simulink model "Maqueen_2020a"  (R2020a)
settings: Solver=VariableStepAuto  StartTime=0.0  StopTime=2  RelTol=1e-3
model workspace: external: MAT-File (data not in the file)
undefined symbols (not defined in the file or in its folder): deg, kg, m, mm, N, rad, s, smiData, X, Y, Z
libraries: sm_lib x459, fl_lib x12, nesl_utility x10
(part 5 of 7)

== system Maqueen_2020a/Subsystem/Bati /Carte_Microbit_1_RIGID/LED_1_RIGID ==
  ReferenceFrame : sm_lib/Frames and Transforms/Reference Frame
  Solid : sm_lib/Body Elements/File Solid  ExtGeomFileName=LED_Defaut_sldprt.STL  UnitType=Custom  ExtGeomFileUnits=mm  StepReaderType=HEX  ExportConvexHullGeometry=off  InertiaType=Custom  Mass=smiData.Solid(10).mass  MassUnits=kg  CenterOfMass=smiData.Solid(10).CoM  CenterOfMassUnits=mm  MomentsOfInertia=smiData.Solid(10).MoI  MomentsOfInertiaUnits=kg*mm^2  ProductsOfInertia=smiData.Solid(10).PoI  ProductsOfInertiaUnits=kg*mm^2  BasedOnType=Density  Density=1000  DensityUnits=kg/m^3  DoExposeReferenceFrame=on  SerializedFrames=<Frames/>  GraphicType=FromGeometry  MarkerShape=Sphere  MarkerSize=10  GraphicVisPropType=SimpleVisualProperties  GraphicDiffuseColor=smiData.Solid(10).color  GraphicSpecularColor=[0.5 0.5 0.5 1.0]  GraphicAmbientColor=[0.15 0.15 0.15 1.0]  GraphicEmissiveColor=[0.0 0.0 0.0 1.0]  GraphicShininess=75  GraphicOpacity=smiData.Solid(10).opacity
  F : PMIOPort  Side=Left
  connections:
  ReferenceFrame/RConn1 -- Solid/RConn1 -- F/RConn1

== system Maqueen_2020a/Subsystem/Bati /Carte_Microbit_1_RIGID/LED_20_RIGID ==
  ReferenceFrame : sm_lib/Frames and Transforms/Reference Frame
  Solid : sm_lib/Body Elements/File Solid  ExtGeomFileName=LED_Defaut_sldprt.STL  UnitType=Custom  ExtGeomFileUnits=mm  StepReaderType=HEX  ExportConvexHullGeometry=off  InertiaType=Custom  Mass=smiData.Solid(10).mass  MassUnits=kg  CenterOfMass=smiData.Solid(10).CoM  CenterOfMassUnits=mm  MomentsOfInertia=smiData.Solid(10).MoI  MomentsOfInertiaUnits=kg*mm^2  ProductsOfInertia=smiData.Solid(10).PoI  ProductsOfInertiaUnits=kg*mm^2  BasedOnType=Density  Density=1000  DensityUnits=kg/m^3  DoExposeReferenceFrame=on  SerializedFrames=<Frames/>  GraphicType=FromGeometry  MarkerShape=Sphere  MarkerSize=10  GraphicVisPropType=SimpleVisualProperties  GraphicDiffuseColor=smiData.Solid(10).color  GraphicSpecularColor=[0.5 0.5 0.5 1.0]  GraphicAmbientColor=[0.15 0.15 0.15 1.0]  GraphicEmissiveColor=[0.0 0.0 0.0 1.0]  GraphicShininess=75  GraphicOpacity=smiData.Solid(10).opacity
  F : PMIOPort  Side=Left
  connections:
  ReferenceFrame/RConn1 -- Solid/RConn1 -- F/RConn1

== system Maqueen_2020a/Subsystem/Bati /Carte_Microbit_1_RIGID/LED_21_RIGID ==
  ReferenceFrame : sm_lib/Frames and Transforms/Reference Frame
  Solid : sm_lib/Body Elements/File Solid  ExtGeomFileName=LED_Defaut_sldprt.STL  UnitType=Custom  ExtGeomFileUnits=mm  StepReaderType=HEX  ExportConvexHullGeometry=off  InertiaType=Custom  Mass=smiData.Solid(10).mass  MassUnits=kg  CenterOfMass=smiData.Solid(10).CoM  CenterOfMassUnits=mm  MomentsOfInertia=smiData.Solid(10).MoI  MomentsOfInertiaUnits=kg*mm^2  ProductsOfInertia=smiData.Solid(10).PoI  ProductsOfInertiaUnits=kg*mm^2  BasedOnType=Density  Density=1000  DensityUnits=kg/m^3  DoExposeReferenceFrame=on  SerializedFrames=<Frames/>  GraphicType=FromGeometry  MarkerShape=Sphere  MarkerSize=10  GraphicVisPropType=SimpleVisualProperties  GraphicDiffuseColor=smiData.Solid(10).color  GraphicSpecularColor=[0.5 0.5 0.5 1.0]  GraphicAmbientColor=[0.15 0.15 0.15 1.0]  GraphicEmissiveColor=[0.0 0.0 0.0 1.0]  GraphicShininess=75  GraphicOpacity=smiData.Solid(10).opacity
  F : PMIOPort  Side=Left
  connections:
  ReferenceFrame/RConn1 -- Solid/RConn1 -- F/RConn1

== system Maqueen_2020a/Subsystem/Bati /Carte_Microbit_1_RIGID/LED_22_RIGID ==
  ReferenceFrame : sm_lib/Frames and Transforms/Reference Frame
  Solid : sm_lib/Body Elements/File Solid  ExtGeomFileName=LED_Defaut_sldprt.STL  UnitType=Custom  ExtGeomFileUnits=mm  StepReaderType=HEX  ExportConvexHullGeometry=off  InertiaType=Custom  Mass=smiData.Solid(10).mass  MassUnits=kg  CenterOfMass=smiData.Solid(10).CoM  CenterOfMassUnits=mm  MomentsOfInertia=smiData.Solid(10).MoI  MomentsOfInertiaUnits=kg*mm^2  ProductsOfInertia=smiData.Solid(10).PoI  ProductsOfInertiaUnits=kg*mm^2  BasedOnType=Density  Density=1000  DensityUnits=kg/m^3  DoExposeReferenceFrame=on  SerializedFrames=<Frames/>  GraphicType=FromGeometry  MarkerShape=Sphere  MarkerSize=10  GraphicVisPropType=SimpleVisualProperties  GraphicDiffuseColor=smiData.Solid(10).color  GraphicSpecularColor=[0.5 0.5 0.5 1.0]  GraphicAmbientColor=[0.15 0.15 0.15 1.0]  GraphicEmissiveColor=[0.0 0.0 0.0 1.0]  GraphicShininess=75  GraphicOpacity=smiData.Solid(10).opacity
  F : PMIOPort  Side=Left
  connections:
  ReferenceFrame/RConn1 -- Solid/RConn1 -- F/RConn1

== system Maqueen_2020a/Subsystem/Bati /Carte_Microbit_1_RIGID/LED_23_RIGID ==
  ReferenceFrame : sm_lib/Frames and Transforms/Reference Frame
  Solid : sm_lib/Body Elements/File Solid  ExtGeomFileName=LED_Defaut_sldprt.STL  UnitType=Custom  ExtGeomFileUnits=mm  StepReaderType=HEX  ExportConvexHullGeometry=off  InertiaType=Custom  Mass=smiData.Solid(10).mass  MassUnits=kg  CenterOfMass=smiData.Solid(10).CoM  CenterOfMassUnits=mm  MomentsOfInertia=smiData.Solid(10).MoI  MomentsOfInertiaUnits=kg*mm^2  ProductsOfInertia=smiData.Solid(10).PoI  ProductsOfInertiaUnits=kg*mm^2  BasedOnType=Density  Density=1000  DensityUnits=kg/m^3  DoExposeReferenceFrame=on  SerializedFrames=<Frames/>  GraphicType=FromGeometry  MarkerShape=Sphere  MarkerSize=10  GraphicVisPropType=SimpleVisualProperties  GraphicDiffuseColor=smiData.Solid(10).color  GraphicSpecularColor=[0.5 0.5 0.5 1.0]  GraphicAmbientColor=[0.15 0.15 0.15 1.0]  GraphicEmissiveColor=[0.0 0.0 0.0 1.0]  GraphicShininess=75  GraphicOpacity=smiData.Solid(10).opacity
  F : PMIOPort  Side=Left
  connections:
  ReferenceFrame/RConn1 -- Solid/RConn1 -- F/RConn1

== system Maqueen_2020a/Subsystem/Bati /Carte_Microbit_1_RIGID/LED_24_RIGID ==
  ReferenceFrame : sm_lib/Frames and Transforms/Reference Frame
  Solid : sm_lib/Body Elements/File Solid  ExtGeomFileName=LED_Defaut_sldprt.STL  UnitType=Custom  ExtGeomFileUnits=mm  StepReaderType=HEX  ExportConvexHullGeometry=off  InertiaType=Custom  Mass=smiData.Solid(10).mass  MassUnits=kg  CenterOfMass=smiData.Solid(10).CoM  CenterOfMassUnits=mm  MomentsOfInertia=smiData.Solid(10).MoI  MomentsOfInertiaUnits=kg*mm^2  ProductsOfInertia=smiData.Solid(10).PoI  ProductsOfInertiaUnits=kg*mm^2  BasedOnType=Density  Density=1000  DensityUnits=kg/m^3  DoExposeReferenceFrame=on  SerializedFrames=<Frames/>  GraphicType=FromGeometry  MarkerShape=Sphere  MarkerSize=10  GraphicVisPropType=SimpleVisualProperties  GraphicDiffuseColor=smiData.Solid(10).color  GraphicSpecularColor=[0.5 0.5 0.5 1.0]  GraphicAmbientColor=[0.15 0.15 0.15 1.0]  GraphicEmissiveColor=[0.0 0.0 0.0 1.0]  GraphicShininess=75  GraphicOpacity=smiData.Solid(10).opacity
  F : PMIOPort  Side=Left
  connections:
  ReferenceFrame/RConn1 -- Solid/RConn1 -- F/RConn1

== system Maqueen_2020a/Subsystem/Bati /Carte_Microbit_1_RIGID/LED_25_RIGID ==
  ReferenceFrame : sm_lib/Frames and Transforms/Reference Frame
  Solid : sm_lib/Body Elements/File Solid  ExtGeomFileName=LED_Defaut_sldprt.STL  UnitType=Custom  ExtGeomFileUnits=mm  StepReaderType=HEX  ExportConvexHullGeometry=off  InertiaType=Custom  Mass=smiData.Solid(10).mass  MassUnits=kg  CenterOfMass=smiData.Solid(10).CoM  CenterOfMassUnits=mm  MomentsOfInertia=smiData.Solid(10).MoI  MomentsOfInertiaUnits=kg*mm^2  ProductsOfInertia=smiData.Solid(10).PoI  ProductsOfInertiaUnits=kg*mm^2  BasedOnType=Density  Density=1000  DensityUnits=kg/m^3  DoExposeReferenceFrame=on  SerializedFrames=<Frames/>  GraphicType=FromGeometry  MarkerShape=Sphere  MarkerSize=10  GraphicVisPropType=SimpleVisualProperties  GraphicDiffuseColor=smiData.Solid(10).color  GraphicSpecularColor=[0.5 0.5 0.5 1.0]  GraphicAmbientColor=[0.15 0.15 0.15 1.0]  GraphicEmissiveColor=[0.0 0.0 0.0 1.0]  GraphicShininess=75  GraphicOpacity=smiData.Solid(10).opacity
  F : PMIOPort  Side=Left
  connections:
  ReferenceFrame/RConn1 -- Solid/RConn1 -- F/RConn1

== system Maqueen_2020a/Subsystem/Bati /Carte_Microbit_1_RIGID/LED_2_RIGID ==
  ReferenceFrame : sm_lib/Frames and Transforms/Reference Frame
  Solid : sm_lib/Body Elements/File Solid  ExtGeomFileName=LED_Defaut_sldprt.STL  UnitType=Custom  ExtGeomFileUnits=mm  StepReaderType=HEX  ExportConvexHullGeometry=off  InertiaType=Custom  Mass=smiData.Solid(10).mass  MassUnits=kg  CenterOfMass=smiData.Solid(10).CoM  CenterOfMassUnits=mm  MomentsOfInertia=smiData.Solid(10).MoI  MomentsOfInertiaUnits=kg*mm^2  ProductsOfInertia=smiData.Solid(10).PoI  ProductsOfInertiaUnits=kg*mm^2  BasedOnType=Density  Density=1000  DensityUnits=kg/m^3  DoExposeReferenceFrame=on  SerializedFrames=<Frames/>  GraphicType=FromGeometry  MarkerShape=Sphere  MarkerSize=10  GraphicVisPropType=SimpleVisualProperties  GraphicDiffuseColor=smiData.Solid(10).color  GraphicSpecularColor=[0.5 0.5 0.5 1.0]  GraphicAmbientColor=[0.15 0.15 0.15 1.0]  GraphicEmissiveColor=[0.0 0.0 0.0 1.0]  GraphicShininess=75  GraphicOpacity=smiData.Solid(10).opacity
  F : PMIOPort  Side=Left
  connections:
  ReferenceFrame/RConn1 -- Solid/RConn1 -- F/RConn1

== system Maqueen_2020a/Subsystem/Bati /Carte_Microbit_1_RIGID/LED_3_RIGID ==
  ReferenceFrame : sm_lib/Frames and Transforms/Reference Frame
  Solid : sm_lib/Body Elements/File Solid  ExtGeomFileName=LED_Defaut_sldprt.STL  UnitType=Custom  ExtGeomFileUnits=mm  StepReaderType=HEX  ExportConvexHullGeometry=off  InertiaType=Custom  Mass=smiData.Solid(10).mass  MassUnits=kg  CenterOfMass=smiData.Solid(10).CoM  CenterOfMassUnits=mm  MomentsOfInertia=smiData.Solid(10).MoI  MomentsOfInertiaUnits=kg*mm^2  ProductsOfInertia=smiData.Solid(10).PoI  ProductsOfInertiaUnits=kg*mm^2  BasedOnType=Density  Density=1000  DensityUnits=kg/m^3  DoExposeReferenceFrame=on  SerializedFrames=<Frames/>  GraphicType=FromGeometry  MarkerShape=Sphere  MarkerSize=10  GraphicVisPropType=SimpleVisualProperties  GraphicDiffuseColor=smiData.Solid(10).color  GraphicSpecularColor=[0.5 0.5 0.5 1.0]  GraphicAmbientColor=[0.15 0.15 0.15 1.0]  GraphicEmissiveColor=[0.0 0.0 0.0 1.0]  GraphicShininess=75  GraphicOpacity=smiData.Solid(10).opacity
  F : PMIOPort  Side=Left
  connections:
  ReferenceFrame/RConn1 -- Solid/RConn1 -- F/RConn1

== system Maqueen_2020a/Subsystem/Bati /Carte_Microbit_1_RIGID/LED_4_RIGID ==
  ReferenceFrame : sm_lib/Frames and Transforms/Reference Frame
  Solid : sm_lib/Body Elements/File Solid  ExtGeomFileName=LED_Defaut_sldprt.STL  UnitType=Custom  ExtGeomFileUnits=mm  StepReaderType=HEX  ExportConvexHullGeometry=off  InertiaType=Custom  Mass=smiData.Solid(10).mass  MassUnits=kg  CenterOfMass=smiData.Solid(10).CoM  CenterOfMassUnits=mm  MomentsOfInertia=smiData.Solid(10).MoI  MomentsOfInertiaUnits=kg*mm^2  ProductsOfInertia=smiData.Solid(10).PoI  ProductsOfInertiaUnits=kg*mm^2  BasedOnType=Density  Density=1000  DensityUnits=kg/m^3  DoExposeReferenceFrame=on  SerializedFrames=<Frames/>  GraphicType=FromGeometry  MarkerShape=Sphere  MarkerSize=10  GraphicVisPropType=SimpleVisualProperties  GraphicDiffuseColor=smiData.Solid(10).color  GraphicSpecularColor=[0.5 0.5 0.5 1.0]  GraphicAmbientColor=[0.15 0.15 0.15 1.0]  GraphicEmissiveColor=[0.0 0.0 0.0 1.0]  GraphicShininess=75  GraphicOpacity=smiData.Solid(10).opacity
  F : PMIOPort  Side=Left
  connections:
  ReferenceFrame/RConn1 -- Solid/RConn1 -- F/RConn1

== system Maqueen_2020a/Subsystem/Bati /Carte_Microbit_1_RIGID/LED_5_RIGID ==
  ReferenceFrame : sm_lib/Frames and Transforms/Reference Frame
  Solid : sm_lib/Body Elements/File Solid  ExtGeomFileName=LED_Defaut_sldprt.STL  UnitType=Custom  ExtGeomFileUnits=mm  StepReaderType=HEX  ExportConvexHullGeometry=off  InertiaType=Custom  Mass=smiData.Solid(10).mass  MassUnits=kg  CenterOfMass=smiData.Solid(10).CoM  CenterOfMassUnits=mm  MomentsOfInertia=smiData.Solid(10).MoI  MomentsOfInertiaUnits=kg*mm^2  ProductsOfInertia=smiData.Solid(10).PoI  ProductsOfInertiaUnits=kg*mm^2  BasedOnType=Density  Density=1000  DensityUnits=kg/m^3  DoExposeReferenceFrame=on  SerializedFrames=<Frames/>  GraphicType=FromGeometry  MarkerShape=Sphere  MarkerSize=10  GraphicVisPropType=SimpleVisualProperties  GraphicDiffuseColor=smiData.Solid(10).color  GraphicSpecularColor=[0.5 0.5 0.5 1.0]  GraphicAmbientColor=[0.15 0.15 0.15 1.0]  GraphicEmissiveColor=[0.0 0.0 0.0 1.0]  GraphicShininess=75  GraphicOpacity=smiData.Solid(10).opacity
  F : PMIOPort  Side=Left
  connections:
  ReferenceFrame/RConn1 -- Solid/RConn1 -- F/RConn1

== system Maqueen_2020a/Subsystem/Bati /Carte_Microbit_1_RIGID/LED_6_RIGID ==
  ReferenceFrame : sm_lib/Frames and Transforms/Reference Frame
  Solid : sm_lib/Body Elements/File Solid  ExtGeomFileName=LED_Defaut_sldprt.STL  UnitType=Custom  ExtGeomFileUnits=mm  StepReaderType=HEX  ExportConvexHullGeometry=off  InertiaType=Custom  Mass=smiData.Solid(10).mass  MassUnits=kg  CenterOfMass=smiData.Solid(10).CoM  CenterOfMassUnits=mm  MomentsOfInertia=smiData.Solid(10).MoI  MomentsOfInertiaUnits=kg*mm^2  ProductsOfInertia=smiData.Solid(10).PoI  ProductsOfInertiaUnits=kg*mm^2  BasedOnType=Density  Density=1000  DensityUnits=kg/m^3  DoExposeReferenceFrame=on  SerializedFrames=<Frames/>  GraphicType=FromGeometry  MarkerShape=Sphere  MarkerSize=10  GraphicVisPropType=SimpleVisualProperties  GraphicDiffuseColor=smiData.Solid(10).color  GraphicSpecularColor=[0.5 0.5 0.5 1.0]  GraphicAmbientColor=[0.15 0.15 0.15 1.0]  GraphicEmissiveColor=[0.0 0.0 0.0 1.0]  GraphicShininess=75  GraphicOpacity=smiData.Solid(10).opacity
  F : PMIOPort  Side=Left
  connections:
  ReferenceFrame/RConn1 -- Solid/RConn1 -- F/RConn1

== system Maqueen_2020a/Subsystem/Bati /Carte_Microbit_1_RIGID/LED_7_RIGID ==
  ReferenceFrame : sm_lib/Frames and Transforms/Reference Frame
  Solid : sm_lib/Body Elements/File Solid  ExtGeomFileName=LED_Defaut_sldprt.STL  UnitType=Custom  ExtGeomFileUnits=mm  StepReaderType=HEX  ExportConvexHullGeometry=off  InertiaType=Custom  Mass=smiData.Solid(10).mass  MassUnits=kg  CenterOfMass=smiData.Solid(10).CoM  CenterOfMassUnits=mm  MomentsOfInertia=smiData.Solid(10).MoI  MomentsOfInertiaUnits=kg*mm^2  ProductsOfInertia=smiData.Solid(10).PoI  ProductsOfInertiaUnits=kg*mm^2  BasedOnType=Density  Density=1000  DensityUnits=kg/m^3  DoExposeReferenceFrame=on  SerializedFrames=<Frames/>  GraphicType=FromGeometry  MarkerShape=Sphere  MarkerSize=10  GraphicVisPropType=SimpleVisualProperties  GraphicDiffuseColor=smiData.Solid(10).color  GraphicSpecularColor=[0.5 0.5 0.5 1.0]  GraphicAmbientColor=[0.15 0.15 0.15 1.0]  GraphicEmissiveColor=[0.0 0.0 0.0 1.0]  GraphicShininess=75  GraphicOpacity=smiData.Solid(10).opacity
  F : PMIOPort  Side=Left
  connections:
  ReferenceFrame/RConn1 -- Solid/RConn1 -- F/RConn1

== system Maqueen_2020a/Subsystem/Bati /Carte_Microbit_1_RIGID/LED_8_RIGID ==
  ReferenceFrame : sm_lib/Frames and Transforms/Reference Frame
  Solid : sm_lib/Body Elements/File Solid  ExtGeomFileName=LED_Defaut_sldprt.STL  UnitType=Custom  ExtGeomFileUnits=mm  StepReaderType=HEX  ExportConvexHullGeometry=off  InertiaType=Custom  Mass=smiData.Solid(10).mass  MassUnits=kg  CenterOfMass=smiData.Solid(10).CoM  CenterOfMassUnits=mm  MomentsOfInertia=smiData.Solid(10).MoI  MomentsOfInertiaUnits=kg*mm^2  ProductsOfInertia=smiData.Solid(10).PoI  ProductsOfInertiaUnits=kg*mm^2  BasedOnType=Density  Density=1000  DensityUnits=kg/m^3  DoExposeReferenceFrame=on  SerializedFrames=<Frames/>  GraphicType=FromGeometry  MarkerShape=Sphere  MarkerSize=10  GraphicVisPropType=SimpleVisualProperties  GraphicDiffuseColor=smiData.Solid(10).color  GraphicSpecularColor=[0.5 0.5 0.5 1.0]  GraphicAmbientColor=[0.15 0.15 0.15 1.0]  GraphicEmissiveColor=[0.0 0.0 0.0 1.0]  GraphicShininess=75  GraphicOpacity=smiData.Solid(10).opacity
  F : PMIOPort  Side=Left
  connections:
  ReferenceFrame/RConn1 -- Solid/RConn1 -- F/RConn1

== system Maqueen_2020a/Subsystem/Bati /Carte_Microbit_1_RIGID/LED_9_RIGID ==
  ReferenceFrame : sm_lib/Frames and Transforms/Reference Frame
  Solid : sm_lib/Body Elements/File Solid  ExtGeomFileName=LED_Defaut_sldprt.STL  UnitType=Custom  ExtGeomFileUnits=mm  StepReaderType=HEX  ExportConvexHullGeometry=off  InertiaType=Custom  Mass=smiData.Solid(10).mass  MassUnits=kg  CenterOfMass=smiData.Solid(10).CoM  CenterOfMassUnits=mm  MomentsOfInertia=smiData.Solid(10).MoI  MomentsOfInertiaUnits=kg*mm^2  ProductsOfInertia=smiData.Solid(10).PoI  ProductsOfInertiaUnits=kg*mm^2  BasedOnType=Density  Density=1000  DensityUnits=kg/m^3  DoExposeReferenceFrame=on  SerializedFrames=<Frames/>  GraphicType=FromGeometry  MarkerShape=Sphere  MarkerSize=10  GraphicVisPropType=SimpleVisualProperties  GraphicDiffuseColor=smiData.Solid(10).color  GraphicSpecularColor=[0.5 0.5 0.5 1.0]  GraphicAmbientColor=[0.15 0.15 0.15 1.0]  GraphicEmissiveColor=[0.0 0.0 0.0 1.0]  GraphicShininess=75  GraphicOpacity=smiData.Solid(10).opacity
  F : PMIOPort  Side=Left
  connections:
  ReferenceFrame/RConn1 -- Solid/RConn1 -- F/RConn1

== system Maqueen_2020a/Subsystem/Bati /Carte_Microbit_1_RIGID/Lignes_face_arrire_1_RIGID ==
  ReferenceFrame : sm_lib/Frames and Transforms/Reference Frame
  Solid : sm_lib/Body Elements/File Solid  ExtGeomFileName=Lignes face arriere_Defaut_sldprt.STL  UnitType=Custom  ExtGeomFileUnits=mm  StepReaderType=HEX  ExportConvexHullGeometry=off  InertiaType=Custom  Mass=smiData.Solid(20).mass  MassUnits=kg  CenterOfMass=smiData.Solid(20).CoM  CenterOfMassUnits=mm  MomentsOfInertia=smiData.Solid(20).MoI  MomentsOfInertiaUnits=kg*mm^2  ProductsOfInertia=smiData.Solid(20).PoI  ProductsOfInertiaUnits=kg*mm^2  BasedOnType=Density  Density=1000  DensityUnits=kg/m^3  DoExposeReferenceFrame=on  SerializedFrames=<Frames/>  GraphicType=FromGeometry  MarkerShape=Sphere  MarkerSize=10  GraphicVisPropType=SimpleVisualProperties  GraphicDiffuseColor=smiData.Solid(20).color  GraphicSpecularColor=[0.5 0.5 0.5 1.0]  GraphicAmbientColor=[0.15 0.15 0.15 1.0]  GraphicEmissiveColor=[0.0 0.0 0.0 1.0]  GraphicShininess=75  GraphicOpacity=smiData.Solid(20).opacity
  F : PMIOPort  Side=Left
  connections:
  ReferenceFrame/RConn1 -- Solid/RConn1 -- F/RConn1

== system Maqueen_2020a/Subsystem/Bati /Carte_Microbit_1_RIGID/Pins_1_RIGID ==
  ReferenceFrame : sm_lib/Frames and Transforms/Reference Frame
  Solid : sm_lib/Body Elements/File Solid  ExtGeomFileName=Pins_Defaut_sldprt.STL  UnitType=Custom  ExtGeomFileUnits=mm  StepReaderType=HEX  ExportConvexHullGeometry=off  InertiaType=Custom  Mass=smiData.Solid(27).mass  MassUnits=kg  CenterOfMass=smiData.Solid(27).CoM  CenterOfMassUnits=mm  MomentsOfInertia=smiData.Solid(27).MoI  MomentsOfInertiaUnits=kg*mm^2  ProductsOfInertia=smiData.Solid(27).PoI  ProductsOfInertiaUnits=kg*mm^2  BasedOnType=Density  Density=1000  DensityUnits=kg/m^3  DoExposeReferenceFrame=on  SerializedFrames=<Frames/>  GraphicType=FromGeometry  MarkerShape=Sphere  MarkerSize=10  GraphicVisPropType=SimpleVisualProperties  GraphicDiffuseColor=smiData.Solid(27).color  GraphicSpecularColor=[0.5 0.5 0.5 1.0]  GraphicAmbientColor=[0.15 0.15 0.15 1.0]  GraphicEmissiveColor=[0.0 0.0 0.0 1.0]  GraphicShininess=75  GraphicOpacity=smiData.Solid(27).opacity
  F : PMIOPort  Side=Left
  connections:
  ReferenceFrame/RConn1 -- Solid/RConn1 -- F/RConn1

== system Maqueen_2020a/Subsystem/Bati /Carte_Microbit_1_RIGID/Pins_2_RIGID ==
  ReferenceFrame : sm_lib/Frames and Transforms/Reference Frame
  Solid : sm_lib/Body Elements/File Solid  ExtGeomFileName=Pins_Defaut_sldprt.STL  UnitType=Custom  ExtGeomFileUnits=mm  StepReaderType=HEX  ExportConvexHullGeometry=off  InertiaType=Custom  Mass=smiData.Solid(27).mass  MassUnits=kg  CenterOfMass=smiData.Solid(27).CoM  CenterOfMassUnits=mm  MomentsOfInertia=smiData.Solid(27).MoI  MomentsOfInertiaUnits=kg*mm^2  ProductsOfInertia=smiData.Solid(27).PoI  ProductsOfInertiaUnits=kg*mm^2  BasedOnType=Density  Density=1000  DensityUnits=kg/m^3  DoExposeReferenceFrame=on  SerializedFrames=<Frames/>  GraphicType=FromGeometry  MarkerShape=Sphere  MarkerSize=10  GraphicVisPropType=SimpleVisualProperties  GraphicDiffuseColor=smiData.Solid(27).color  GraphicSpecularColor=[0.5 0.5 0.5 1.0]  GraphicAmbientColor=[0.15 0.15 0.15 1.0]  GraphicEmissiveColor=[0.0 0.0 0.0 1.0]  GraphicShininess=75  GraphicOpacity=smiData.Solid(27).opacity
  F : PMIOPort  Side=Left
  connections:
  ReferenceFrame/RConn1 -- Solid/RConn1 -- F/RConn1

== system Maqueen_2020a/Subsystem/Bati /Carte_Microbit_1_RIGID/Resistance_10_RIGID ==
  ReferenceFrame : sm_lib/Frames and Transforms/Reference Frame
  Solid : sm_lib/Body Elements/File Solid  ExtGeomFileName=Resistance_Defaut_sldprt.STL  UnitType=Custom  ExtGeomFileUnits=mm  StepReaderType=HEX  ExportConvexHullGeometry=off  InertiaType=Custom  Mass=smiData.Solid(7).mass  MassUnits=kg  CenterOfMass=smiData.Solid(7).CoM  CenterOfMassUnits=mm  MomentsOfInertia=smiData.Solid(7).MoI  MomentsOfInertiaUnits=kg*mm^2  ProductsOfInertia=smiData.Solid(7).PoI  ProductsOfInertiaUnits=kg*mm^2  BasedOnType=Density  Density=1000  DensityUnits=kg/m^3  DoExposeReferenceFrame=on  SerializedFrames=<Frames/>  GraphicType=FromGeometry  MarkerShape=Sphere  MarkerSize=10  GraphicVisPropType=SimpleVisualProperties  GraphicDiffuseColor=smiData.Solid(7).color  GraphicSpecularColor=[0.5 0.5 0.5 1.0]  GraphicAmbientColor=[0.15 0.15 0.15 1.0]  GraphicEmissiveColor=[0.0 0.0 0.0 1.0]  GraphicShininess=75  GraphicOpacity=smiData.Solid(7).opacity
  F : PMIOPort  Side=Left
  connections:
  ReferenceFrame/RConn1 -- Solid/RConn1 -- F/RConn1

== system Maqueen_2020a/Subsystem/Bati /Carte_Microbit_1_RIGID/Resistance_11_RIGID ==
  ReferenceFrame : sm_lib/Frames and Transforms/Reference Frame
  Solid : sm_lib/Body Elements/File Solid  ExtGeomFileName=Resistance_Defaut_sldprt.STL  UnitType=Custom  ExtGeomFileUnits=mm  StepReaderType=HEX  ExportConvexHullGeometry=off  InertiaType=Custom  Mass=smiData.Solid(7).mass  MassUnits=kg  CenterOfMass=smiData.Solid(7).CoM  CenterOfMassUnits=mm  MomentsOfInertia=smiData.Solid(7).MoI  MomentsOfInertiaUnits=kg*mm^2  ProductsOfInertia=smiData.Solid(7).PoI  ProductsOfInertiaUnits=kg*mm^2  BasedOnType=Density  Density=1000  DensityUnits=kg/m^3  DoExposeReferenceFrame=on  SerializedFrames=<Frames/>  GraphicType=FromGeometry  MarkerShape=Sphere  MarkerSize=10  GraphicVisPropType=SimpleVisualProperties  GraphicDiffuseColor=smiData.Solid(7).color  GraphicSpecularColor=[0.5 0.5 0.5 1.0]  GraphicAmbientColor=[0.15 0.15 0.15 1.0]  GraphicEmissiveColor=[0.0 0.0 0.0 1.0]  GraphicShininess=75  GraphicOpacity=smiData.Solid(7).opacity
  F : PMIOPort  Side=Left
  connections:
  ReferenceFrame/RConn1 -- Solid/RConn1 -- F/RConn1

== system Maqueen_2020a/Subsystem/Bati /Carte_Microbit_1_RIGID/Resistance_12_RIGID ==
  ReferenceFrame : sm_lib/Frames and Transforms/Reference Frame
  Solid : sm_lib/Body Elements/File Solid  ExtGeomFileName=Resistance_Defaut_sldprt.STL  UnitType=Custom  ExtGeomFileUnits=mm  StepReaderType=HEX  ExportConvexHullGeometry=off  InertiaType=Custom  Mass=smiData.Solid(7).mass  MassUnits=kg  CenterOfMass=smiData.Solid(7).CoM  CenterOfMassUnits=mm  MomentsOfInertia=smiData.Solid(7).MoI  MomentsOfInertiaUnits=kg*mm^2  ProductsOfInertia=smiData.Solid(7).PoI  ProductsOfInertiaUnits=kg*mm^2  BasedOnType=Density  Density=1000  DensityUnits=kg/m^3  DoExposeReferenceFrame=on  SerializedFrames=<Frames/>  GraphicType=FromGeometry  MarkerShape=Sphere  MarkerSize=10  GraphicVisPropType=SimpleVisualProperties  GraphicDiffuseColor=smiData.Solid(7).color  GraphicSpecularColor=[0.5 0.5 0.5 1.0]  GraphicAmbientColor=[0.15 0.15 0.15 1.0]  GraphicEmissiveColor=[0.0 0.0 0.0 1.0]  GraphicShininess=75  GraphicOpacity=smiData.Solid(7).opacity
  F : PMIOPort  Side=Left
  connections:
  ReferenceFrame/RConn1 -- Solid/RConn1 -- F/RConn1

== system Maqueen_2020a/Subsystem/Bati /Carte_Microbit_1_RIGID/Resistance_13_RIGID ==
  ReferenceFrame : sm_lib/Frames and Transforms/Reference Frame
  Solid : sm_lib/Body Elements/File Solid  ExtGeomFileName=Resistance_Defaut_sldprt.STL  UnitType=Custom  ExtGeomFileUnits=mm  StepReaderType=HEX  ExportConvexHullGeometry=off  InertiaType=Custom  Mass=smiData.Solid(7).mass  MassUnits=kg  CenterOfMass=smiData.Solid(7).CoM  CenterOfMassUnits=mm  MomentsOfInertia=smiData.Solid(7).MoI  MomentsOfInertiaUnits=kg*mm^2  ProductsOfInertia=smiData.Solid(7).PoI  ProductsOfInertiaUnits=kg*mm^2  BasedOnType=Density  Density=1000  DensityUnits=kg/m^3  DoExposeReferenceFrame=on  SerializedFrames=<Frames/>  GraphicType=FromGeometry  MarkerShape=Sphere  MarkerSize=10  GraphicVisPropType=SimpleVisualProperties  GraphicDiffuseColor=smiData.Solid(7).color  GraphicSpecularColor=[0.5 0.5 0.5 1.0]  GraphicAmbientColor=[0.15 0.15 0.15 1.0]  GraphicEmissiveColor=[0.0 0.0 0.0 1.0]  GraphicShininess=75  GraphicOpacity=smiData.Solid(7).opacity
  F : PMIOPort  Side=Left
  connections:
  ReferenceFrame/RConn1 -- Solid/RConn1 -- F/RConn1

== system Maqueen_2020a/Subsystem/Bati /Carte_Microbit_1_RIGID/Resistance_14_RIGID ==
  ReferenceFrame : sm_lib/Frames and Transforms/Reference Frame
  Solid : sm_lib/Body Elements/File Solid  ExtGeomFileName=Resistance_Defaut_sldprt.STL  UnitType=Custom  ExtGeomFileUnits=mm  StepReaderType=HEX  ExportConvexHullGeometry=off  InertiaType=Custom  Mass=smiData.Solid(7).mass  MassUnits=kg  CenterOfMass=smiData.Solid(7).CoM  CenterOfMassUnits=mm  MomentsOfInertia=smiData.Solid(7).MoI  MomentsOfInertiaUnits=kg*mm^2  ProductsOfInertia=smiData.Solid(7).PoI  ProductsOfInertiaUnits=kg*mm^2  BasedOnType=Density  Density=1000  DensityUnits=kg/m^3  DoExposeReferenceFrame=on  SerializedFrames=<Frames/>  GraphicType=FromGeometry  MarkerShape=Sphere  MarkerSize=10  GraphicVisPropType=SimpleVisualProperties  GraphicDiffuseColor=smiData.Solid(7).color  GraphicSpecularColor=[0.5 0.5 0.5 1.0]  GraphicAmbientColor=[0.15 0.15 0.15 1.0]  GraphicEmissiveColor=[0.0 0.0 0.0 1.0]  GraphicShininess=75  GraphicOpacity=smiData.Solid(7).opacity
  F : PMIOPort  Side=Left
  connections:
  ReferenceFrame/RConn1 -- Solid/RConn1 -- F/RConn1

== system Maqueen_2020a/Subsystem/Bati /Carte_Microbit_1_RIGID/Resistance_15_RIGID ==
  ReferenceFrame : sm_lib/Frames and Transforms/Reference Frame
  Solid : sm_lib/Body Elements/File Solid  ExtGeomFileName=Resistance_Defaut_sldprt.STL  UnitType=Custom  ExtGeomFileUnits=mm  StepReaderType=HEX  ExportConvexHullGeometry=off  InertiaType=Custom  Mass=smiData.Solid(7).mass  MassUnits=kg  CenterOfMass=smiData.Solid(7).CoM  CenterOfMassUnits=mm  MomentsOfInertia=smiData.Solid(7).MoI  MomentsOfInertiaUnits=kg*mm^2  ProductsOfInertia=smiData.Solid(7).PoI  ProductsOfInertiaUnits=kg*mm^2  BasedOnType=Density  Density=1000  DensityUnits=kg/m^3  DoExposeReferenceFrame=on  SerializedFrames=<Frames/>  GraphicType=FromGeometry  MarkerShape=Sphere  MarkerSize=10  GraphicVisPropType=SimpleVisualProperties  GraphicDiffuseColor=smiData.Solid(7).color  GraphicSpecularColor=[0.5 0.5 0.5 1.0]  GraphicAmbientColor=[0.15 0.15 0.15 1.0]  GraphicEmissiveColor=[0.0 0.0 0.0 1.0]  GraphicShininess=75  GraphicOpacity=smiData.Solid(7).opacity
  F : PMIOPort  Side=Left
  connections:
  ReferenceFrame/RConn1 -- Solid/RConn1 -- F/RConn1

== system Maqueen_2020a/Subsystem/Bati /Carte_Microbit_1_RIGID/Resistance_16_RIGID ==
  ReferenceFrame : sm_lib/Frames and Transforms/Reference Frame
  Solid : sm_lib/Body Elements/File Solid  ExtGeomFileName=Resistance_Defaut_sldprt.STL  UnitType=Custom  ExtGeomFileUnits=mm  StepReaderType=HEX  ExportConvexHullGeometry=off  InertiaType=Custom  Mass=smiData.Solid(7).mass  MassUnits=kg  CenterOfMass=smiData.Solid(7).CoM  CenterOfMassUnits=mm  MomentsOfInertia=smiData.Solid(7).MoI  MomentsOfInertiaUnits=kg*mm^2  ProductsOfInertia=smiData.Solid(7).PoI  ProductsOfInertiaUnits=kg*mm^2  BasedOnType=Density  Density=1000  DensityUnits=kg/m^3  DoExposeReferenceFrame=on  SerializedFrames=<Frames/>  GraphicType=FromGeometry  MarkerShape=Sphere  MarkerSize=10  GraphicVisPropType=SimpleVisualProperties  GraphicDiffuseColor=smiData.Solid(7).color  GraphicSpecularColor=[0.5 0.5 0.5 1.0]  GraphicAmbientColor=[0.15 0.15 0.15 1.0]  GraphicEmissiveColor=[0.0 0.0 0.0 1.0]  GraphicShininess=75  GraphicOpacity=smiData.Solid(7).opacity
  F : PMIOPort  Side=Left
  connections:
  ReferenceFrame/RConn1 -- Solid/RConn1 -- F/RConn1

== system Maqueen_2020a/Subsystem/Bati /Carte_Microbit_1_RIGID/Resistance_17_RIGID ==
  ReferenceFrame : sm_lib/Frames and Transforms/Reference Frame
  Solid : sm_lib/Body Elements/File Solid  ExtGeomFileName=Resistance_Defaut_sldprt.STL  UnitType=Custom  ExtGeomFileUnits=mm  StepReaderType=HEX  ExportConvexHullGeometry=off  InertiaType=Custom  Mass=smiData.Solid(7).mass  MassUnits=kg  CenterOfMass=smiData.Solid(7).CoM  CenterOfMassUnits=mm  MomentsOfInertia=smiData.Solid(7).MoI  MomentsOfInertiaUnits=kg*mm^2  ProductsOfInertia=smiData.Solid(7).PoI  ProductsOfInertiaUnits=kg*mm^2  BasedOnType=Density  Density=1000  DensityUnits=kg/m^3  DoExposeReferenceFrame=on  SerializedFrames=<Frames/>  GraphicType=FromGeometry  MarkerShape=Sphere  MarkerSize=10  GraphicVisPropType=SimpleVisualProperties  GraphicDiffuseColor=smiData.Solid(7).color  GraphicSpecularColor=[0.5 0.5 0.5 1.0]  GraphicAmbientColor=[0.15 0.15 0.15 1.0]  GraphicEmissiveColor=[0.0 0.0 0.0 1.0]  GraphicShininess=75  GraphicOpacity=smiData.Solid(7).opacity
  F : PMIOPort  Side=Left
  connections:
  ReferenceFrame/RConn1 -- Solid/RConn1 -- F/RConn1

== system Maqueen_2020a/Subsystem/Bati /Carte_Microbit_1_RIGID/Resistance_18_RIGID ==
  ReferenceFrame : sm_lib/Frames and Transforms/Reference Frame
  Solid : sm_lib/Body Elements/File Solid  ExtGeomFileName=Resistance_Defaut_sldprt.STL  UnitType=Custom  ExtGeomFileUnits=mm  StepReaderType=HEX  ExportConvexHullGeometry=off  InertiaType=Custom  Mass=smiData.Solid(7).mass  MassUnits=kg  CenterOfMass=smiData.Solid(7).CoM  CenterOfMassUnits=mm  MomentsOfInertia=smiData.Solid(7).MoI  MomentsOfInertiaUnits=kg*mm^2  ProductsOfInertia=smiData.Solid(7).PoI  ProductsOfInertiaUnits=kg*mm^2  BasedOnType=Density  Density=1000  DensityUnits=kg/m^3  DoExposeReferenceFrame=on  SerializedFrames=<Frames/>  GraphicType=FromGeometry  MarkerShape=Sphere  MarkerSize=10  GraphicVisPropType=SimpleVisualProperties  GraphicDiffuseColor=smiData.Solid(7).color  GraphicSpecularColor=[0.5 0.5 0.5 1.0]  GraphicAmbientColor=[0.15 0.15 0.15 1.0]  GraphicEmissiveColor=[0.0 0.0 0.0 1.0]  GraphicShininess=75  GraphicOpacity=smiData.Solid(7).opacity
  F : PMIOPort  Side=Left
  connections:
  ReferenceFrame/RConn1 -- Solid/RConn1 -- F/RConn1

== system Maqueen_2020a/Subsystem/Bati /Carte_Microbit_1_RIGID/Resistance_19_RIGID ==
  ReferenceFrame : sm_lib/Frames and Transforms/Reference Frame
  Solid : sm_lib/Body Elements/File Solid  ExtGeomFileName=Resistance_Defaut_sldprt.STL  UnitType=Custom  ExtGeomFileUnits=mm  StepReaderType=HEX  ExportConvexHullGeometry=off  InertiaType=Custom  Mass=smiData.Solid(7).mass  MassUnits=kg  CenterOfMass=smiData.Solid(7).CoM  CenterOfMassUnits=mm  MomentsOfInertia=smiData.Solid(7).MoI  MomentsOfInertiaUnits=kg*mm^2  ProductsOfInertia=smiData.Solid(7).PoI  ProductsOfInertiaUnits=kg*mm^2  BasedOnType=Density  Density=1000  DensityUnits=kg/m^3  DoExposeReferenceFrame=on  SerializedFrames=<Frames/>  GraphicType=FromGeometry  MarkerShape=Sphere  MarkerSize=10  GraphicVisPropType=SimpleVisualProperties  GraphicDiffuseColor=smiData.Solid(7).color  GraphicSpecularColor=[0.5 0.5 0.5 1.0]  GraphicAmbientColor=[0.15 0.15 0.15 1.0]  GraphicEmissiveColor=[0.0 0.0 0.0 1.0]  GraphicShininess=75  GraphicOpacity=smiData.Solid(7).opacity
  F : PMIOPort  Side=Left
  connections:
  ReferenceFrame/RConn1 -- Solid/RConn1 -- F/RConn1

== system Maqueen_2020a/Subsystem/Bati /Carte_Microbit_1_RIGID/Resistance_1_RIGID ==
  ReferenceFrame : sm_lib/Frames and Transforms/Reference Frame
  Solid : sm_lib/Body Elements/File Solid  ExtGeomFileName=Resistance_Defaut_sldprt.STL  UnitType=Custom  ExtGeomFileUnits=mm  StepReaderType=HEX  ExportConvexHullGeometry=off  InertiaType=Custom  Mass=smiData.Solid(7).mass  MassUnits=kg  CenterOfMass=smiData.Solid(7).CoM  CenterOfMassUnits=mm  MomentsOfInertia=smiData.Solid(7).MoI  MomentsOfInertiaUnits=kg*mm^2  ProductsOfInertia=smiData.Solid(7).PoI  ProductsOfInertiaUnits=kg*mm^2  BasedOnType=Density  Density=1000  DensityUnits=kg/m^3  DoExposeReferenceFrame=on  SerializedFrames=<Frames/>  GraphicType=FromGeometry  MarkerShape=Sphere  MarkerSize=10  GraphicVisPropType=SimpleVisualProperties  GraphicDiffuseColor=smiData.Solid(7).color  GraphicSpecularColor=[0.5 0.5 0.5 1.0]  GraphicAmbientColor=[0.15 0.15 0.15 1.0]  GraphicEmissiveColor=[0.0 0.0 0.0 1.0]  GraphicShininess=75  GraphicOpacity=smiData.Solid(7).opacity
  F : PMIOPort  Side=Left
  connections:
  ReferenceFrame/RConn1 -- Solid/RConn1 -- F/RConn1

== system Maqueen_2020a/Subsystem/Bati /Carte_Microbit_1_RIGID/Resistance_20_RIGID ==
  ReferenceFrame : sm_lib/Frames and Transforms/Reference Frame
  Solid : sm_lib/Body Elements/File Solid  ExtGeomFileName=Resistance_Defaut_sldprt.STL  UnitType=Custom  ExtGeomFileUnits=mm  StepReaderType=HEX  ExportConvexHullGeometry=off  InertiaType=Custom  Mass=smiData.Solid(7).mass  MassUnits=kg  CenterOfMass=smiData.Solid(7).CoM  CenterOfMassUnits=mm  MomentsOfInertia=smiData.Solid(7).MoI  MomentsOfInertiaUnits=kg*mm^2  ProductsOfInertia=smiData.Solid(7).PoI  ProductsOfInertiaUnits=kg*mm^2  BasedOnType=Density  Density=1000  DensityUnits=kg/m^3  DoExposeReferenceFrame=on  SerializedFrames=<Frames/>  GraphicType=FromGeometry  MarkerShape=Sphere  MarkerSize=10  GraphicVisPropType=SimpleVisualProperties  GraphicDiffuseColor=smiData.Solid(7).color  GraphicSpecularColor=[0.5 0.5 0.5 1.0]  GraphicAmbientColor=[0.15 0.15 0.15 1.0]  GraphicEmissiveColor=[0.0 0.0 0.0 1.0]  GraphicShininess=75  GraphicOpacity=smiData.Solid(7).opacity
  F : PMIOPort  Side=Left
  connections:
  ReferenceFrame/RConn1 -- Solid/RConn1 -- F/RConn1

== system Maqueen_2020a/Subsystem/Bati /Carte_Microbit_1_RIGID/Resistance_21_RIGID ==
  ReferenceFrame : sm_lib/Frames and Transforms/Reference Frame
  Solid : sm_lib/Body Elements/File Solid  ExtGeomFileName=Resistance_Defaut_sldprt.STL  UnitType=Custom  ExtGeomFileUnits=mm  StepReaderType=HEX  ExportConvexHullGeometry=off  InertiaType=Custom  Mass=smiData.Solid(7).mass  MassUnits=kg  CenterOfMass=smiData.Solid(7).CoM  CenterOfMassUnits=mm  MomentsOfInertia=smiData.Solid(7).MoI  MomentsOfInertiaUnits=kg*mm^2  ProductsOfInertia=smiData.Solid(7).PoI  ProductsOfInertiaUnits=kg*mm^2  BasedOnType=Density  Density=1000  DensityUnits=kg/m^3  DoExposeReferenceFrame=on  SerializedFrames=<Frames/>  GraphicType=FromGeometry  MarkerShape=Sphere  MarkerSize=10  GraphicVisPropType=SimpleVisualProperties  GraphicDiffuseColor=smiData.Solid(7).color  GraphicSpecularColor=[0.5 0.5 0.5 1.0]  GraphicAmbientColor=[0.15 0.15 0.15 1.0]  GraphicEmissiveColor=[0.0 0.0 0.0 1.0]  GraphicShininess=75  GraphicOpacity=smiData.Solid(7).opacity
  F : PMIOPort  Side=Left
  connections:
  ReferenceFrame/RConn1 -- Solid/RConn1 -- F/RConn1

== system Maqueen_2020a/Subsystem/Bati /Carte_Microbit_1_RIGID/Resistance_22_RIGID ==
  ReferenceFrame : sm_lib/Frames and Transforms/Reference Frame
  Solid : sm_lib/Body Elements/File Solid  ExtGeomFileName=Resistance_Defaut_sldprt.STL  UnitType=Custom  ExtGeomFileUnits=mm  StepReaderType=HEX  ExportConvexHullGeometry=off  InertiaType=Custom  Mass=smiData.Solid(7).mass  MassUnits=kg  CenterOfMass=smiData.Solid(7).CoM  CenterOfMassUnits=mm  MomentsOfInertia=smiData.Solid(7).MoI  MomentsOfInertiaUnits=kg*mm^2  ProductsOfInertia=smiData.Solid(7).PoI  ProductsOfInertiaUnits=kg*mm^2  BasedOnType=Density  Density=1000  DensityUnits=kg/m^3  DoExposeReferenceFrame=on  SerializedFrames=<Frames/>  GraphicType=FromGeometry  MarkerShape=Sphere  MarkerSize=10  GraphicVisPropType=SimpleVisualProperties  GraphicDiffuseColor=smiData.Solid(7).color  GraphicSpecularColor=[0.5 0.5 0.5 1.0]  GraphicAmbientColor=[0.15 0.15 0.15 1.0]  GraphicEmissiveColor=[0.0 0.0 0.0 1.0]  GraphicShininess=75  GraphicOpacity=smiData.Solid(7).opacity
  F : PMIOPort  Side=Left
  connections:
  ReferenceFrame/RConn1 -- Solid/RConn1 -- F/RConn1

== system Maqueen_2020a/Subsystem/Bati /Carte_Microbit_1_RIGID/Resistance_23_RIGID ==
  ReferenceFrame : sm_lib/Frames and Transforms/Reference Frame
  Solid : sm_lib/Body Elements/File Solid  ExtGeomFileName=Resistance_Defaut_sldprt.STL  UnitType=Custom  ExtGeomFileUnits=mm  StepReaderType=HEX  ExportConvexHullGeometry=off  InertiaType=Custom  Mass=smiData.Solid(7).mass  MassUnits=kg  CenterOfMass=smiData.Solid(7).CoM  CenterOfMassUnits=mm  MomentsOfInertia=smiData.Solid(7).MoI  MomentsOfInertiaUnits=kg*mm^2  ProductsOfInertia=smiData.Solid(7).PoI  ProductsOfInertiaUnits=kg*mm^2  BasedOnType=Density  Density=1000  DensityUnits=kg/m^3  DoExposeReferenceFrame=on  SerializedFrames=<Frames/>  GraphicType=FromGeometry  MarkerShape=Sphere  MarkerSize=10  GraphicVisPropType=SimpleVisualProperties  GraphicDiffuseColor=smiData.Solid(7).color  GraphicSpecularColor=[0.5 0.5 0.5 1.0]  GraphicAmbientColor=[0.15 0.15 0.15 1.0]  GraphicEmissiveColor=[0.0 0.0 0.0 1.0]  GraphicShininess=75  GraphicOpacity=smiData.Solid(7).opacity
  F : PMIOPort  Side=Left
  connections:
  ReferenceFrame/RConn1 -- Solid/RConn1 -- F/RConn1

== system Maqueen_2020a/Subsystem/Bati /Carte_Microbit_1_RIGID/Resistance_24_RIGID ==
  ReferenceFrame : sm_lib/Frames and Transforms/Reference Frame
  Solid : sm_lib/Body Elements/File Solid  ExtGeomFileName=Resistance_Defaut_sldprt.STL  UnitType=Custom  ExtGeomFileUnits=mm  StepReaderType=HEX  ExportConvexHullGeometry=off  InertiaType=Custom  Mass=smiData.Solid(7).mass  MassUnits=kg  CenterOfMass=smiData.Solid(7).CoM  CenterOfMassUnits=mm  MomentsOfInertia=smiData.Solid(7).MoI  MomentsOfInertiaUnits=kg*mm^2  ProductsOfInertia=smiData.Solid(7).PoI  ProductsOfInertiaUnits=kg*mm^2  BasedOnType=Density  Density=1000  DensityUnits=kg/m^3  DoExposeReferenceFrame=on  SerializedFrames=<Frames/>  GraphicType=FromGeometry  MarkerShape=Sphere  MarkerSize=10  GraphicVisPropType=SimpleVisualProperties  GraphicDiffuseColor=smiData.Solid(7).color  GraphicSpecularColor=[0.5 0.5 0.5 1.0]  GraphicAmbientColor=[0.15 0.15 0.15 1.0]  GraphicEmissiveColor=[0.0 0.0 0.0 1.0]  GraphicShininess=75  GraphicOpacity=smiData.Solid(7).opacity
  F : PMIOPort  Side=Left
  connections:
  ReferenceFrame/RConn1 -- Solid/RConn1 -- F/RConn1

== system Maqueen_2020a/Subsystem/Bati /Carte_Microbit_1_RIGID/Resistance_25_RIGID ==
  ReferenceFrame : sm_lib/Frames and Transforms/Reference Frame
  Solid : sm_lib/Body Elements/File Solid  ExtGeomFileName=Resistance_Defaut_sldprt.STL  UnitType=Custom  ExtGeomFileUnits=mm  StepReaderType=HEX  ExportConvexHullGeometry=off  InertiaType=Custom  Mass=smiData.Solid(7).mass  MassUnits=kg  CenterOfMass=smiData.Solid(7).CoM  CenterOfMassUnits=mm  MomentsOfInertia=smiData.Solid(7).MoI  MomentsOfInertiaUnits=kg*mm^2  ProductsOfInertia=smiData.Solid(7).PoI  ProductsOfInertiaUnits=kg*mm^2  BasedOnType=Density  Density=1000  DensityUnits=kg/m^3  DoExposeReferenceFrame=on  SerializedFrames=<Frames/>  GraphicType=FromGeometry  MarkerShape=Sphere  MarkerSize=10  GraphicVisPropType=SimpleVisualProperties  GraphicDiffuseColor=smiData.Solid(7).color  GraphicSpecularColor=[0.5 0.5 0.5 1.0]  GraphicAmbientColor=[0.15 0.15 0.15 1.0]  GraphicEmissiveColor=[0.0 0.0 0.0 1.0]  GraphicShininess=75  GraphicOpacity=smiData.Solid(7).opacity
  F : PMIOPort  Side=Left
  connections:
  ReferenceFrame/RConn1 -- Solid/RConn1 -- F/RConn1

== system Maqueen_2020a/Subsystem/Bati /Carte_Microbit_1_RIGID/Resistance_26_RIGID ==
  ReferenceFrame : sm_lib/Frames and Transforms/Reference Frame
  Solid : sm_lib/Body Elements/File Solid  ExtGeomFileName=Resistance_Defaut_sldprt.STL  UnitType=Custom  ExtGeomFileUnits=mm  StepReaderType=HEX  ExportConvexHullGeometry=off  InertiaType=Custom  Mass=smiData.Solid(7).mass  MassUnits=kg  CenterOfMass=smiData.Solid(7).CoM  CenterOfMassUnits=mm  MomentsOfInertia=smiData.Solid(7).MoI  MomentsOfInertiaUnits=kg*mm^2  ProductsOfInertia=smiData.Solid(7).PoI  ProductsOfInertiaUnits=kg*mm^2  BasedOnType=Density  Density=1000  DensityUnits=kg/m^3  DoExposeReferenceFrame=on  SerializedFrames=<Frames/>  GraphicType=FromGeometry  MarkerShape=Sphere  MarkerSize=10  GraphicVisPropType=SimpleVisualProperties  GraphicDiffuseColor=smiData.Solid(7).color  GraphicSpecularColor=[0.5 0.5 0.5 1.0]  GraphicAmbientColor=[0.15 0.15 0.15 1.0]  GraphicEmissiveColor=[0.0 0.0 0.0 1.0]  GraphicShininess=75  GraphicOpacity=smiData.Solid(7).opacity
  F : PMIOPort  Side=Left
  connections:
  ReferenceFrame/RConn1 -- Solid/RConn1 -- F/RConn1

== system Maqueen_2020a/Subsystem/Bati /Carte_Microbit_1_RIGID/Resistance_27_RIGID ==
  ReferenceFrame : sm_lib/Frames and Transforms/Reference Frame
  Solid : sm_lib/Body Elements/File Solid  ExtGeomFileName=Resistance_Defaut_sldprt.STL  UnitType=Custom  ExtGeomFileUnits=mm  StepReaderType=HEX  ExportConvexHullGeometry=off  InertiaType=Custom  Mass=smiData.Solid(7).mass  MassUnits=kg  CenterOfMass=smiData.Solid(7).CoM  CenterOfMassUnits=mm  MomentsOfInertia=smiData.Solid(7).MoI  MomentsOfInertiaUnits=kg*mm^2  ProductsOfInertia=smiData.Solid(7).PoI  ProductsOfInertiaUnits=kg*mm^2  BasedOnType=Density  Density=1000  DensityUnits=kg/m^3  DoExposeReferenceFrame=on  SerializedFrames=<Frames/>  GraphicType=FromGeometry  MarkerShape=Sphere  MarkerSize=10  GraphicVisPropType=SimpleVisualProperties  GraphicDiffuseColor=smiData.Solid(7).color  GraphicSpecularColor=[0.5 0.5 0.5 1.0]  GraphicAmbientColor=[0.15 0.15 0.15 1.0]  GraphicEmissiveColor=[0.0 0.0 0.0 1.0]  GraphicShininess=75  GraphicOpacity=smiData.Solid(7).opacity
  F : PMIOPort  Side=Left
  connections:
  ReferenceFrame/RConn1 -- Solid/RConn1 -- F/RConn1

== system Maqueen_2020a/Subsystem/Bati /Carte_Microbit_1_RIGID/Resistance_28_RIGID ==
  ReferenceFrame : sm_lib/Frames and Transforms/Reference Frame
  Solid : sm_lib/Body Elements/File Solid  ExtGeomFileName=Resistance_Defaut_sldprt.STL  UnitType=Custom  ExtGeomFileUnits=mm  StepReaderType=HEX  ExportConvexHullGeometry=off  InertiaType=Custom  Mass=smiData.Solid(7).mass  MassUnits=kg  CenterOfMass=smiData.Solid(7).CoM  CenterOfMassUnits=mm  MomentsOfInertia=smiData.Solid(7).MoI  MomentsOfInertiaUnits=kg*mm^2  ProductsOfInertia=smiData.Solid(7).PoI  ProductsOfInertiaUnits=kg*mm^2  BasedOnType=Density  Density=1000  DensityUnits=kg/m^3  DoExposeReferenceFrame=on  SerializedFrames=<Frames/>  GraphicType=FromGeometry  MarkerShape=Sphere  MarkerSize=10  GraphicVisPropType=SimpleVisualProperties  GraphicDiffuseColor=smiData.Solid(7).color  GraphicSpecularColor=[0.5 0.5 0.5 1.0]  GraphicAmbientColor=[0.15 0.15 0.15 1.0]  GraphicEmissiveColor=[0.0 0.0 0.0 1.0]  GraphicShininess=75  GraphicOpacity=smiData.Solid(7).opacity
  F : PMIOPort  Side=Left
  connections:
  ReferenceFrame/RConn1 -- Solid/RConn1 -- F/RConn1

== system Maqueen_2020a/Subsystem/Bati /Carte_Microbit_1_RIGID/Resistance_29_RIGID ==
  ReferenceFrame : sm_lib/Frames and Transforms/Reference Frame
  Solid : sm_lib/Body Elements/File Solid  ExtGeomFileName=Resistance_Defaut_sldprt.STL  UnitType=Custom  ExtGeomFileUnits=mm  StepReaderType=HEX  ExportConvexHullGeometry=off  InertiaType=Custom  Mass=smiData.Solid(7).mass  MassUnits=kg  CenterOfMass=smiData.Solid(7).CoM  CenterOfMassUnits=mm  MomentsOfInertia=smiData.Solid(7).MoI  MomentsOfInertiaUnits=kg*mm^2  ProductsOfInertia=smiData.Solid(7).PoI  ProductsOfInertiaUnits=kg*mm^2  BasedOnType=Density  Density=1000  DensityUnits=kg/m^3  DoExposeReferenceFrame=on  SerializedFrames=<Frames/>  GraphicType=FromGeometry  MarkerShape=Sphere  MarkerSize=10  GraphicVisPropType=SimpleVisualProperties  GraphicDiffuseColor=smiData.Solid(7).color  GraphicSpecularColor=[0.5 0.5 0.5 1.0]  GraphicAmbientColor=[0.15 0.15 0.15 1.0]  GraphicEmissiveColor=[0.0 0.0 0.0 1.0]  GraphicShininess=75  GraphicOpacity=smiData.Solid(7).opacity
  F : PMIOPort  Side=Left
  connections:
  ReferenceFrame/RConn1 -- Solid/RConn1 -- F/RConn1

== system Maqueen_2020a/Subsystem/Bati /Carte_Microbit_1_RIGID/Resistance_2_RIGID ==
  ReferenceFrame : sm_lib/Frames and Transforms/Reference Frame
  Solid : sm_lib/Body Elements/File Solid  ExtGeomFileName=Resistance_Defaut_sldprt.STL  UnitType=Custom  ExtGeomFileUnits=mm  StepReaderType=HEX  ExportConvexHullGeometry=off  InertiaType=Custom  Mass=smiData.Solid(7).mass  MassUnits=kg  CenterOfMass=smiData.Solid(7).CoM  CenterOfMassUnits=mm  MomentsOfInertia=smiData.Solid(7).MoI  MomentsOfInertiaUnits=kg*mm^2  ProductsOfInertia=smiData.Solid(7).PoI  ProductsOfInertiaUnits=kg*mm^2  BasedOnType=Density  Density=1000  DensityUnits=kg/m^3  DoExposeReferenceFrame=on  SerializedFrames=<Frames/>  GraphicType=FromGeometry  MarkerShape=Sphere  MarkerSize=10  GraphicVisPropType=SimpleVisualProperties  GraphicDiffuseColor=smiData.Solid(7).color  GraphicSpecularColor=[0.5 0.5 0.5 1.0]  GraphicAmbientColor=[0.15 0.15 0.15 1.0]  GraphicEmissiveColor=[0.0 0.0 0.0 1.0]  GraphicShininess=75  GraphicOpacity=smiData.Solid(7).opacity
  F : PMIOPort  Side=Left
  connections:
  ReferenceFrame/RConn1 -- Solid/RConn1 -- F/RConn1

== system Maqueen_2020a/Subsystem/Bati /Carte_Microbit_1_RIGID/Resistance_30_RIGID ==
  ReferenceFrame : sm_lib/Frames and Transforms/Reference Frame
  Solid : sm_lib/Body Elements/File Solid  ExtGeomFileName=Resistance_Defaut_sldprt.STL  UnitType=Custom  ExtGeomFileUnits=mm  StepReaderType=HEX  ExportConvexHullGeometry=off  InertiaType=Custom  Mass=smiData.Solid(7).mass  MassUnits=kg  CenterOfMass=smiData.Solid(7).CoM  CenterOfMassUnits=mm  MomentsOfInertia=smiData.Solid(7).MoI  MomentsOfInertiaUnits=kg*mm^2  ProductsOfInertia=smiData.Solid(7).PoI  ProductsOfInertiaUnits=kg*mm^2  BasedOnType=Density  Density=1000  DensityUnits=kg/m^3  DoExposeReferenceFrame=on  SerializedFrames=<Frames/>  GraphicType=FromGeometry  MarkerShape=Sphere  MarkerSize=10  GraphicVisPropType=SimpleVisualProperties  GraphicDiffuseColor=smiData.Solid(7).color  GraphicSpecularColor=[0.5 0.5 0.5 1.0]  GraphicAmbientColor=[0.15 0.15 0.15 1.0]  GraphicEmissiveColor=[0.0 0.0 0.0 1.0]  GraphicShininess=75  GraphicOpacity=smiData.Solid(7).opacity
  F : PMIOPort  Side=Left
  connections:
  ReferenceFrame/RConn1 -- Solid/RConn1 -- F/RConn1

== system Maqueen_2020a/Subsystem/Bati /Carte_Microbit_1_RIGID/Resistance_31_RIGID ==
  ReferenceFrame : sm_lib/Frames and Transforms/Reference Frame
  Solid : sm_lib/Body Elements/File Solid  ExtGeomFileName=Resistance_Defaut_sldprt.STL  UnitType=Custom  ExtGeomFileUnits=mm  StepReaderType=HEX  ExportConvexHullGeometry=off  InertiaType=Custom  Mass=smiData.Solid(7).mass  MassUnits=kg  CenterOfMass=smiData.Solid(7).CoM  CenterOfMassUnits=mm  MomentsOfInertia=smiData.Solid(7).MoI  MomentsOfInertiaUnits=kg*mm^2  ProductsOfInertia=smiData.Solid(7).PoI  ProductsOfInertiaUnits=kg*mm^2  BasedOnType=Density  Density=1000  DensityUnits=kg/m^3  DoExposeReferenceFrame=on  SerializedFrames=<Frames/>  GraphicType=FromGeometry  MarkerShape=Sphere  MarkerSize=10  GraphicVisPropType=SimpleVisualProperties  GraphicDiffuseColor=smiData.Solid(7).color  GraphicSpecularColor=[0.5 0.5 0.5 1.0]  GraphicAmbientColor=[0.15 0.15 0.15 1.0]  GraphicEmissiveColor=[0.0 0.0 0.0 1.0]  GraphicShininess=75  GraphicOpacity=smiData.Solid(7).opacity
  F : PMIOPort  Side=Left
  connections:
  ReferenceFrame/RConn1 -- Solid/RConn1 -- F/RConn1

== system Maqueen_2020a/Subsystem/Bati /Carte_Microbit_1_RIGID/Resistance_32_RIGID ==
  ReferenceFrame : sm_lib/Frames and Transforms/Reference Frame
  Solid : sm_lib/Body Elements/File Solid  ExtGeomFileName=Resistance_Defaut_sldprt.STL  UnitType=Custom  ExtGeomFileUnits=mm  StepReaderType=HEX  ExportConvexHullGeometry=off  InertiaType=Custom  Mass=smiData.Solid(7).mass  MassUnits=kg  CenterOfMass=smiData.Solid(7).CoM  CenterOfMassUnits=mm  MomentsOfInertia=smiData.Solid(7).MoI  MomentsOfInertiaUnits=kg*mm^2  ProductsOfInertia=smiData.Solid(7).PoI  ProductsOfInertiaUnits=kg*mm^2  BasedOnType=Density  Density=1000  DensityUnits=kg/m^3  DoExposeReferenceFrame=on  SerializedFrames=<Frames/>  GraphicType=FromGeometry  MarkerShape=Sphere  MarkerSize=10  GraphicVisPropType=SimpleVisualProperties  GraphicDiffuseColor=smiData.Solid(7).color  GraphicSpecularColor=[0.5 0.5 0.5 1.0]  GraphicAmbientColor=[0.15 0.15 0.15 1.0]  GraphicEmissiveColor=[0.0 0.0 0.0 1.0]  GraphicShininess=75  GraphicOpacity=smiData.Solid(7).opacity
  F : PMIOPort  Side=Left
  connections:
  ReferenceFrame/RConn1 -- Solid/RConn1 -- F/RConn1

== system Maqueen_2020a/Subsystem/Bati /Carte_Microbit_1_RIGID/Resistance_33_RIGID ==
  ReferenceFrame : sm_lib/Frames and Transforms/Reference Frame
  Solid : sm_lib/Body Elements/File Solid  ExtGeomFileName=Resistance_Defaut_sldprt.STL  UnitType=Custom  ExtGeomFileUnits=mm  StepReaderType=HEX  ExportConvexHullGeometry=off  InertiaType=Custom  Mass=smiData.Solid(7).mass  MassUnits=kg  CenterOfMass=smiData.Solid(7).CoM  CenterOfMassUnits=mm  MomentsOfInertia=smiData.Solid(7).MoI  MomentsOfInertiaUnits=kg*mm^2  ProductsOfInertia=smiData.Solid(7).PoI  ProductsOfInertiaUnits=kg*mm^2  BasedOnType=Density  Density=1000  DensityUnits=kg/m^3  DoExposeReferenceFrame=on  SerializedFrames=<Frames/>  GraphicType=FromGeometry  MarkerShape=Sphere  MarkerSize=10  GraphicVisPropType=SimpleVisualProperties  GraphicDiffuseColor=smiData.Solid(7).color  GraphicSpecularColor=[0.5 0.5 0.5 1.0]  GraphicAmbientColor=[0.15 0.15 0.15 1.0]  GraphicEmissiveColor=[0.0 0.0 0.0 1.0]  GraphicShininess=75  GraphicOpacity=smiData.Solid(7).opacity
  F : PMIOPort  Side=Left
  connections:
  ReferenceFrame/RConn1 -- Solid/RConn1 -- F/RConn1
